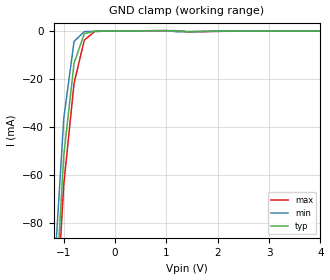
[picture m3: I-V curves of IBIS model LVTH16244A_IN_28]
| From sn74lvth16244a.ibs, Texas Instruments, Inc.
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|   Model LVTH16244A Input_IN_28
[Model]   LVTH16244A_IN_28
Model_type  Input
Polarity   Inverting
Vinl = 0.8V
Vinh = 2.0V
| variable   typ   min   max
C_comp   4pf   NA   NA
[Temperature Range]   40   -25   100
| Ambient temperature   25   -40   85
[Voltage range]   2.8   2.7   2.9
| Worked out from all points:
|   GND clamp passes 1 mA (typ) near -0.58 V on its own axis
[GND Clamp]
|   Voltage   I(typ)   I(min)   I(max)
-5V       -2.138A    -2.473A    -1.923A
-1.2V     -126.1mA   -106.1mA   -137mA
-1V       -51.76mA   -36.37mA   -64.02mA
-800mV    -13.38mA   -4.345mA   -21.79mA
-600mV    -1.084mA   -246uA     -3.776mA
-400mV    -92.45uA   -105.6uA   -204.4uA
-200mV    -42.72uA   -51.5uA    -37.72uA
1V        160.8uA    194.8uA    142.1uA
1.2V      124.3uA    -305.5uA   136.2uA
1.4V      -281.4uA   -253.4uA   -297.9uA
5V        -181pA     3.953uA    817.6pA
